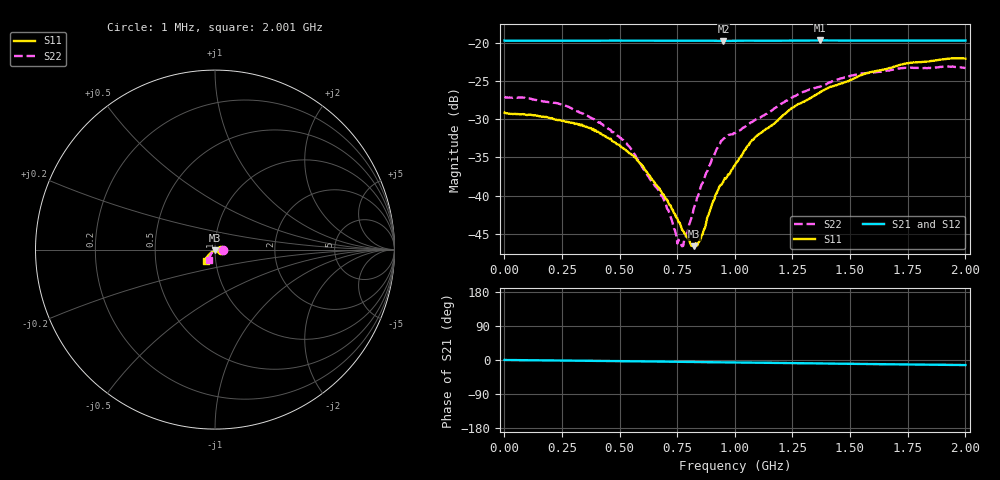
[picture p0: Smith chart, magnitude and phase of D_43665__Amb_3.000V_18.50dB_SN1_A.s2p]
! device id: 43665_
! dir: \\malibu\benchdata\1_engineers\tn_data\43665_75ohm\new\sparar\43665_\amb\3p000v\18p50db
! Serial: 1
! Insertion: A
! Temp: Amb
! VDD: 3.000V
! Attenuation Step: 18.50dB
! IDD: 1.450530e+00mA
! FILE NAME
! DATE 03-27-2009 08:37:53
! CORRECTED  DATA
#  Hz  S  RI  R  75
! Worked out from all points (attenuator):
!   401 points, 1 MHz to 2.001 GHz, reference 75 ohm
!   highest |S21| = -19.65 dB at 1.371 GHz (marker M1); lowest = -19.7 dB at 951 MHz (marker M2)
!   lowest |S11| = -46.6 dB at 821 MHz (marker M3), VSWR 1.01, Z = 75.2 - j0.655 ohm
!   |S11| at or under -10 dB: start of sweep to end of sweep
!   |S22| runs from -46.6 to -23.1 dB; largest |S21 - S12| = 0.0012
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1000000  0.035 -0.000249  0.1041 0.000111  0.1038 -0.000171  0.0445 -0.000555
2.31e8  0.0312 0.00182  0.1037 -0.00241  0.1037 -0.00239  0.0399 0.00552
3.36e8  0.0292 0.00174  0.1036 -0.00358  0.1037 -0.00351  0.0339 0.00715
4.26e8  0.0248 0.00204  0.1037 -0.00451  0.1037 -0.00443  0.0286 0.00663
5.26e8  0.0199 0.00134  0.1036 -0.00578  0.1037 -0.00574  0.0217 0.00478
5.91e8  0.0162 0.000618  0.1035 -0.00653  0.1036 -0.00644  0.0157 0.0038
6.71e8  0.0112 -0.00107  0.1036 -0.0074  0.1036 -0.00729  0.0106 0.000382
7.06e8  0.00926 -0.00178  0.1036 -0.00784  0.1036 -0.00773  0.00816 -0.000848
7.61e8  0.00589 -0.00306  0.1036 -0.00862  0.1036 -0.00846  0.00356 -0.00326
7.81e8  0.00454 -0.00341  0.1035 -0.00888  0.1036 -0.00874  0.0019 -0.0048
8.21e8  0.00167 -0.00435  0.1035 -0.00947  0.1035 -0.00934  -0.00128 -0.00803
8.51e8  -0.000329 -0.00514  0.1034 -0.00996  0.1034 -0.00979  -0.00331 -0.0108
9.11e8  -0.00507 -0.00797  0.103 -0.0108  0.1031 -0.0106  -0.00894 -0.0162
9.51e8  -0.00787 -0.00956  0.1027 -0.0111  0.1028 -0.0109  -0.0153 -0.018
1.001e9  -0.0116 -0.0108  0.1029 -0.0112  0.1029 -0.0111  -0.0191 -0.0171
1.096e9  -0.0193 -0.0154  0.103 -0.0129  0.1031 -0.0126  -0.0214 -0.0234
1.241e9  -0.0289 -0.0228  0.1028 -0.0145  0.103 -0.0143  -0.0264 -0.0342
1.336e9  -0.0341 -0.0283  0.1028 -0.0158  0.1031 -0.0156  -0.0297 -0.0406
1.371e9  -0.0365 -0.0307  0.1028 -0.0164  0.1031 -0.0162  -0.0295 -0.0427
1.511e9  -0.0431 -0.0387  0.1022 -0.0183  0.1026 -0.0181  -0.0338 -0.0514
1.671e9  -0.0486 -0.0486  0.1019 -0.0202  0.1022 -0.0203  -0.0344 -0.0565
2.001e9  -0.0498 -0.0615  0.1011 -0.024  0.1009 -0.0251  -0.0332 -0.06
